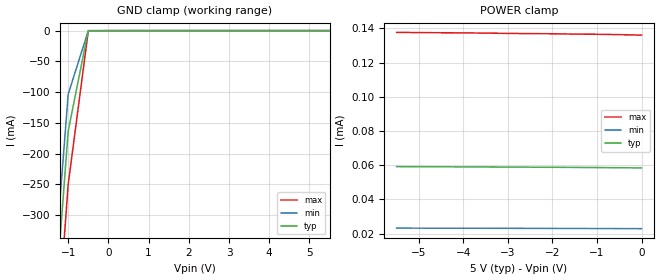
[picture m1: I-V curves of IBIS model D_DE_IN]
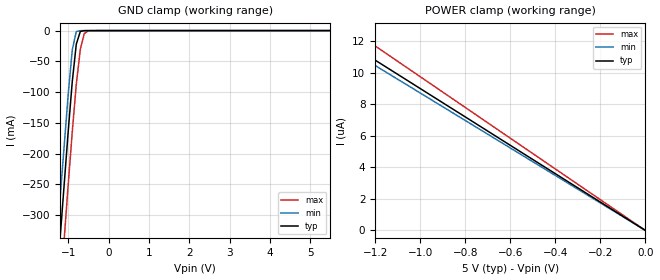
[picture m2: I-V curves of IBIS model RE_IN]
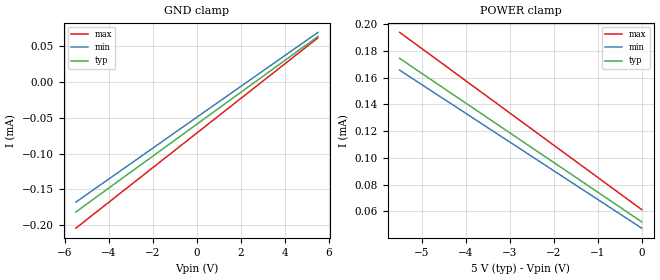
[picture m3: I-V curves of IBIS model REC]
|   Texas Instruments Incorporated
|   Data Transmissions Products
|   IBIS Model for SN65HVD53
|   14D SOIC Package
[IBIS Ver]   3.2
[Comment char]   |_char
[File name]   hvd53.ibs
[File Rev]   1.0
[Date]   4May06
[Source]   File originated at Texas Instruments Incorporated.
   Data Transmission Products Group.
[Notes]
[Disclaimer]
(C) Copyright Texas Instruments Incorporated 2002
   All rights reserved
  Texas Instruments Incorporated hereby grants the user of this IBIS
model a non-exclusive, nontransferable license to use this IBIS model
under the following terms.  Before using this IBIS model, the user
should read this license.  If the user does not accept these terms,
the IBIS model should be returned to Texas Instruments within 30 days.
  The user is granted this license only to use the IBIS model and
is not granted rights to sell, load, rent, lease or license the IBIS
model in whole or in part, or in modified form to anyone other than
user.  User may modify the IBIS model to suit its specific applications
but rights to derivative works and such modifications shall belong to
Texas Instruments.
  This IBIS model is provided on an "AS IS" basis and Texas Instruments
makes absolutely no warranty with respect to the information contained
herein.  TEXAS INSTRUMENTS DISCLAIMS AND CUSTOMER WAIVES ALL WARRANTIES,
EXPRESS OR IMPLIED, INCLUDING WARRANTIES OF MERCHANTABILITY OR FITNESS
FOR A PARTICULAR PURPOSE. The entire risk as to quality and performance
is with the Customer. ACCORDINGLY, IN NO EVENT SHALL THE COMPANY BE LIABLE
FOR ANY DAMAGES, WHETHER IN CONTRACT OR TORT,INCLUDING ANY LOST PROFITS
OR OTHER INCIDENTAL, CONSEQUENTIAL, EXEMPLARY, OR PUNITIVE DAMAGES ARISING
OUT OF THE USE OR APPLICATION OF THE IBIS model provided in this package.
Further, Texas Instruments reserves the right to discontinue or make changes
without notice to any product herein to improve reliability, function, or
design. Texas Instruments does not convey any license under patent rights
or any other intellectual property rights, including those of third parties.
Contact Texas Instruments at ATTN:DATA TRANSMISSIONS
[Copyright]   Copyright 2002, Texas Instruments, All Rights Reserved
[Component]   HVD53D
[Manufacturer]  Texas Instruments Incorporated
[Package]
|   typ   min   max
R_pkg   0.071   0.050   0.091
L_pkg   2.203nH   1.540nH   2.930nH
C_pkg   0.465pF   0.385pF   0.609pF
[Pin]   signal_name   model_name   R_pin   L_pin   C_pin
2   R   RECEIVER_OUT   0.076   2.346n   0.483p
3   RE   RE_IN   0.072   1.934n   0.404p
4   DE   D_DE_IN   0.053   1.585n   0.397p
5   D   D_DE_IN   0.062   1.755n   0.395p
6   GND   GND   0.090   2.593n   0.498p
7   GND   GND   0.072   2.930n   0.608p
9   Y   DRVR   0.073   2.300n   0.480p
10   Z   DRVR   0.076   2.012n   0.407p
11   A   REC   0.070   1.897n   0.412p
12   B   REC   0.050   1.540n   0.385p
13   VCC   POWER   0.091   2.615n   0.500p
14   VCC   POWER   0.073   2.929n   0.609p
[Diff_pin]   inv_pin   vdiff   tdelay_typ   tdelay_min   tdelay_max
| The 'A' pin is Diff_pin and the 'B' pin is the inv_pin
9   10   0.200   0 0 0
11   12   0.200   0 0 0
| Models and submodels in the file (5): D_DE_IN (Input), RE_IN (Input), REC (Input), DRVR (I/O), RECEIVER_OUT (3-state)
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|   Driver Input / Driver Enable / Model
[Model]   D_DE_IN
Model_type   Input
|Signals   D,DE
Vinh = 2.0
Vinl = 0.8
|   typ   min   max
C_comp   23pF   19pF   27pF
|   typ   min   max
[Temperature Range]   27   -40   85
[Voltage range]   5.0V   4.5V   5.5V
[GND_clamp]
|   Voltage   I(typ)   I(min)   I(max)
-5.5V     -3.894A    -3.744A    -4.095A
-1.5V     -596.3mA   -523.6mA   -696.4mA
-1V       -163.5mA   -103.3mA   -250mA
-500mV    -18.38uA   -37.25uA   -400.5uA
5.5V      58.51uA    136uA      22.98uA
[Power_clamp]
| Note that the[POWER_clamp]voltage table is referenced to Vcc
| and is calculated using Vtable=Vcc - Vmeasured.
|   Voltage   I(typ)   I(min)   I(max)
-5.5V     59.15uA    23.21uA    137.6uA
-5V       59.11uA    23.19uA    137.5uA
-4.5V     59.06uA    23.17uA    137.4uA
-4V       59.01uA    23.15uA    137.3uA
-3.5V     58.95uA    23.12uA    137.2uA
-3V       58.9uA     23.1uA     137uA
-2.5V     58.83uA    23.07uA    136.9uA
-2V       58.77uA    23.04uA    136.8uA
-1.5V     58.69uA    23.01uA    136.6uA
-1V       58.61uA    22.98uA    136.5uA
-500mV    58.51uA    22.94uA    136.3uA
0V        58.4uA     22.9uA     136uA
|   Receiver Enable / Model
[Model]   RE_IN
Model_type   Input
|Signals   RE
Vinh = 2.0
Vinl = 0.8
|   typ   min   max
C_comp   23pF   19pF   27pF
|   typ   min   max
[Temperature Range]   27   -40   85
[Voltage range]   5.0V   4.5V   5.5V
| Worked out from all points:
|   GND clamp passes 1 mA (typ) near -0.67 V on its own axis
[GND_clamp]
|   Voltage   I(typ)   I(min)   I(max)
-5.5V     -3.894A    -3.744A    -4.095A
-1.5V     -596.4mA   -523.8mA   -696.5mA
-1V       -163.6mA   -103.4mA   -250.1mA
-900mV    -83.23mA   -31.53mA   -164.7mA
-800mV    -22.17mA   -1.468mA   -87.57mA
-700mV    -1.371mA   -163.6uA   -30.45mA
-600mV    -86.24uA   -88.19uA   -4.747mA
-500mV    -50.55uA   -61.03uA   -417.4uA
5.5V      4.496uA    23.09pA    8.71uA
[Power_clamp]
| Note that the[POWER_clamp]voltage table is referenced to Vcc
| and is calculated using Vtable=Vcc - Vmeasured.
|   Voltage   I(typ)   I(min)   I(max)
-5.5V     49.46uA    47.9uA     53.58uA
-1.6V     14.39uA    13.94uA    15.59uA
-1.4V     12.59uA    12.19uA    13.64uA
-1.2V     10.79uA    10.45uA    11.69uA
0V        0A         0A         0A
|   Receiver Input / Model
[Model]   REC
Model_type   Input
|Signals   A,B
Vinh = 2.0
Vinl = 0.8
|   typ   min   max
C_comp   3pF   2.5pF   3.5pF
|   typ   min   max
[Temperature Range]   27   -40   85
[Voltage range]   5.0V   4.5V   5.5V
[GND_clamp]
|   Voltage   I(typ)   I(min)   I(max)
-5.5V     -181.4uA   -167.7uA   -204uA
-3.5V     -136.8uA   -124.6uA   -155.7uA
1V        -36.71uA   -27.75uA   -47.12uA
5.5V      63.31uA    68.95uA    61.36uA
[Power_clamp]
| Note that the[POWER_clamp]voltage table is referenced to Vcc
| and is calculated using Vtable=Vcc - Vmeasured.
|   Voltage   I(typ)   I(min)   I(max)
-5.5V     174.4uA    165.6uA    193.8uA
-5V       163.2uA    154.8uA    181.8uA
-4.5V     152.1uA    144.1uA    169.8uA
-4V       141uA      133.4uA    157.7uA
-3.5V     129.9uA    122.6uA    145.7uA
-3V       118.8uA    111.9uA    133.6uA
-2.5V     107.7uA    101.2uA    121.6uA
-2V       96.62uA    90.42uA    109.5uA
-1.5V     85.52uA    79.68uA    97.5uA
-1V       74.41uA    68.95uA    85.45uA
-500mV    63.31uA    58.21uA    73.4uA
0V        52.2uA     47.47uA    61.36uA
